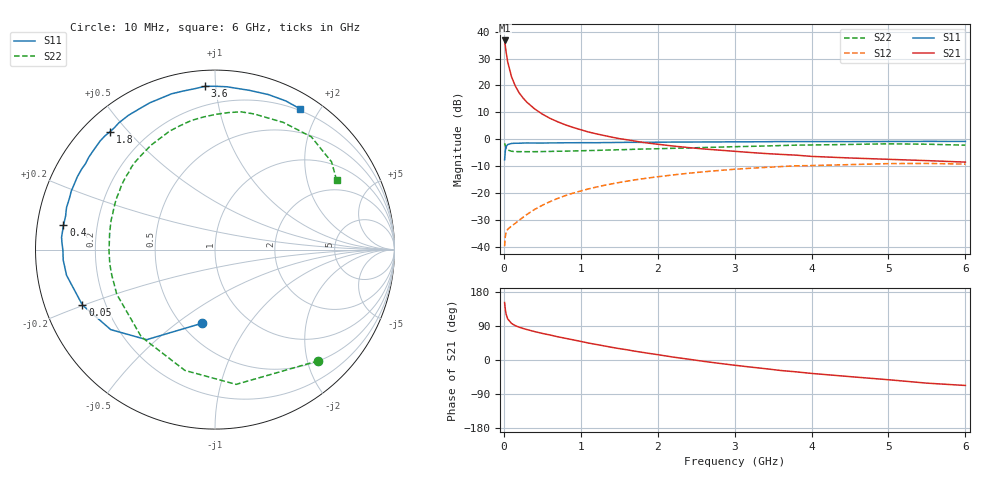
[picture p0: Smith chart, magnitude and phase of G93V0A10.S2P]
! SIEMENS Small Signal Semiconductors
! BFG235
! Si NPN RF Bipolar Junction Transistor in SOT223
! VCE = 3 V  IC = 100 mA
! Common Emitter S-Parameters:  July  1994
# GHz  S  MA  R  50
!  f  S11  S21  S12  S22
! GHz  MAG  ANG  MAG  ANG  MAG  ANG  MAG  ANG
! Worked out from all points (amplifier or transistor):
!   40 points, 10 MHz to 6 GHz, reference 50 ohm
!   highest |S21| = 36.7 dB at 10 MHz (marker M1)
!   |S21| within 3 dB of that: start of sweep to 23.73 MHz
!   unconditionally stable (mu >= 1): 458.8 MHz to 1.507 GHz
!   at 200 MHz: K = 0.79, MSG = 23.6 dB, |S12| = -30.0 dB
!   at 1.5 GHz: K = 1.00, MAG = 8.0 dB, |S12| = -16.0 dB
!   at 6 GHz: K = 0.92, MSG = 0.4 dB, |S12| = -9.2 dB
!   S11 on the Smith chart (normalised r, x): 10 MHz: 0.63, -0.62; 50 MHz: 0.12, -0.20; 400 MHz: 0.08, +0.08; 1.8 GHz: 0.08, +0.45; 3.6 GHz: 0.09, +0.94; 6 GHz: 0.18, +1.76
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0.01  0.4164 -99.9  68.56 151.6  0.0104 62.8  0.8458 -47.1
0.02  0.63 -127.2  53.27 132.5  0.0159 47.6  0.7601 -81.1
0.03  0.7323 -142.5  41.5 120.7  0.0191 40.0  0.6937 -104.0
0.05  0.8007 -157.3  27.48 108.4  0.0214 32.3  0.6363 -130.2
0.1  0.8394 -170.2  14.48 96.5  0.0246 34.8  0.6012 -155.5
0.15  0.8478 -176.1  9.715 90.5  0.0277 40.2  0.5924 -166.0
0.2  0.8472 -179.6  7.266 86.6  0.0318 44.9  0.5916 -171.9
0.25  0.8536 177.4  5.855 83.2  0.0357 48.5  0.59 -176.1
0.3  0.8576 175.4  4.887 80.4  0.0403 51.8  0.5907 -179.5
0.4  0.8549 170.9  3.68 75.0  0.05 54.7  0.5904 175.5
0.5  0.8531 167.3  2.943 70.2  0.0597 56.2  0.594 171.3
0.7  0.86 160.5  2.119 61.3  0.0801 56.0  0.6016 164.1
0.9  0.8648 155.0  1.666 53.2  0.1003 53.5  0.6089 157.8
1.1  0.8678 148.8  1.37 44.7  0.1203 50.3  0.6199 151.7
1.4  0.8734 141.5  1.102 33.6  0.1488 44.6  0.6364 143.3
1.8  0.8793 131.8  0.882 20.2  0.1851 36.2  0.6604 132.3
2.2  0.8902 122.8  0.752 7.7  0.2187 27.2  0.6822 121.5
3.2  0.901 101.5  0.571 -18.5  0.2904 4.1  0.7407 95.4
3.6  0.9115 93.4  0.526 -27.7  0.3122 -5.8  0.7671 84.4
4.5  0.9078 77.7  0.451 -43.9  0.3397 -25.5  0.8045 61.7
5.5  0.9175 64.5  0.403 -61.1  0.3574 -47.2  0.8127 36.9
6  0.9163 58.8  0.378 -67.2  0.3474 -55.4  0.7799 29.7
